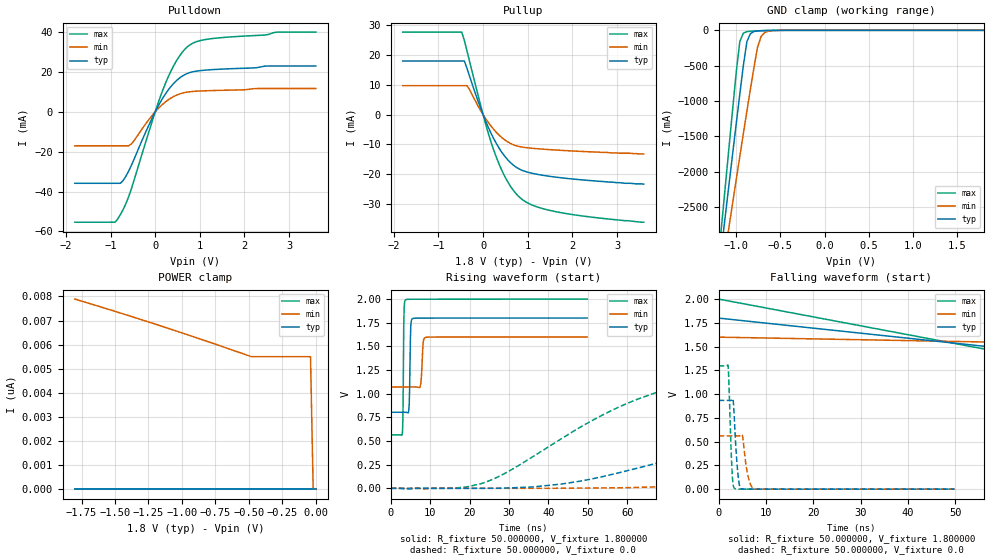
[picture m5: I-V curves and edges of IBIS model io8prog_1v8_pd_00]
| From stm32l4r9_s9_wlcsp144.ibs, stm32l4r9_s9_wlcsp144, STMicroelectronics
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|   Model io8prog_1v8_pd_00
[Model]  io8prog_1v8_pd_00
Model_type I/O
Polarity   Non-Inverting
Enable   Active-Low
Vinl =   0.540000V
Vinh =   1.260000V
Vmeas =  0.900000V
Cref =   100.000000nF
Rref =   1.000000k
Vref =   1.800000V
C_comp   2.197300pF   2.162700pF   2.264100pF
[Temperature Range]   25.000000   0.125000k   -40.000000
[Pullup Reference]   1.800000V   1.600000V   2.000000V
[Pulldown Reference]   0.0V   0.0V   0.0V
[POWER Clamp Reference]   1.800000V   1.600000V   2.000000V
[GND Clamp Reference]   0.0V   0.0V   0.0V
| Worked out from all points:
|   slope of the pulldown table from 0 to 0.27 V, typ, clamps not added: 26.2 ohm
|   slope of the pullup table from 0 to 0.27 V, typ, clamps not added: 30.1 ohm
|   GND clamp passes 1 mA (typ) near -0.58 V on its own axis
|   rising waveform, R_fixture 50.000000, V_fixture 1.800000: 20-80 % time 248ps typ, 382ps min, 184ps max; typ from 0.804 V to 1.8 V
|   rising waveform, R_fixture 50.000000, V_fixture 0.0: 20-80 % time 65.2ns typ, 116ns min, 36.2ns max; typ from 0 V to 0.933 V
|   falling waveform, R_fixture 50.000000, V_fixture 1.800000: 20-80 % time 115ns typ, 165ns min, 91.9ns max; typ from 1.8 V to 0.804 V
|   falling waveform, R_fixture 50.000000, V_fixture 0.0: 20-80 % time 709ps typ, 1.01ns min, 545ps max; typ from 0.933 V to 0 V
[Pulldown]
|Voltage   I(typ)   I(min)   I(max)
-1.8V     -35.82mA   -17.03mA   -55.34mA
-900mV    -35.82mA   -17.03mA   -55.34mA
-840mV    -35.82mA   -17.03mA   -53.76mA
-720mV    -34.49mA   -17.03mA   -49.08mA
-540mV    -27.18mA   -16.22mA   -39.07mA
-60mV     -2.756mA   -1.584mA   -4.226mA
240mV     9.353mA    5.172mA    14.85mA
480mV     15.75mA    8.427mA    25.77mA
720mV     19.29mA    9.947mA    32.62mA
960mV     20.57mA    10.43mA    35.5mA
1.32V     21.27mA    10.74mA    36.91mA
3.6V      23.03mA    11.73mA    40.05mA
[Pullup]
|Voltage   I(typ)   I(min)   I(max)
-1.8V     18.05mA    9.741mA    27.78mA
-480mV    18.05mA    9.741mA    27.78mA
-420mV    18.05mA    9.741mA    25.03mA
-360mV    15.57mA    9.741mA    21.38mA
60mV      -2.268mA   -1.401mA   -3.341mA
240mV     -8.143mA   -5.004mA   -12mA
360mV     -11.31mA   -6.914mA   -16.72mA
540mV     -15mA      -9.056mA   -22.31mA
840mV     -18.52mA   -10.83mA   -28.11mA
1.14V     -19.87mA   -11.38mA   -30.67mA
1.68V     -21.13mA   -11.96mA   -32.81mA
3.6V      -23.4mA    -13.2mA    -36.2mA
[GND_clamp]
|Voltage   I(typ)   I(min)   I(max)
-1.8V     -9.861A    -8.8A      -9.626A
-1.16V    -3.004A    -3.417A    -2.68A
-1.12V    -2.579A    -3.088A    -2.15A
-1.08V    -2.155A    -2.76A     -1.623A
-1V       -1.315A    -2.108A    -586.3mA
-960mV    -900.6mA   -1.784A    -158.3mA
-920mV    -496.8mA   -1.462A    -39.4mA
-880mV    -160.5mA   -1.144A    -17.83mA
-840mV    -45.94mA   -830.4mA   -12.53mA
-760mV    -8.275mA   -243mA     -7.558mA
-680mV    -3.402mA   -33.06mA   -3.844mA
1.8V      47.61uA    51.9uA     39.21uA
[POWER_clamp]
|Voltage   I(typ)   I(min)   I(max)
-1.8V     0A         7.891nA    0A
-1.14V    0A         6.744nA    0A
-480mV    0A         5.5nA      0A
-40mV     0A         5.5nA      0A
-20mV     0A         0A         0A
0V        0A         0A         0A
[Ramp]
| variable   typ   min   max
dV/dt_r  0.56009/65.12327n   0.33637/0.11606u   0.77826/36.16950n
dV/dt_f  0.59737/66.14891n   0.31692/0.11606u   0.86050/35.16380n
R_load = 50.000000
[Rising Waveform]
R_fixture= 50.000000
V_fixture= 1.800000
V_fixture_min= 1.600000
V_fixture_max= 2.000000
|time   V(typ)   V(min)   V(max)
0s        803.6mV    1.071V     565.2mV
2.903ns   803.6mV    1.071V     566.5mV
3.103ns   803.6mV    1.071V     740.3mV
3.403ns   803.6mV    1.071V     1.897V
3.804ns   803.4mV    1.071V     1.992V
4.605ns   827.4mV    1.071V     1.997V
5.105ns   1.718V     1.071V     1.997V
5.606ns   1.794V     1.071V     1.998V
8.809ns   1.798V     1.594V     1.998V
49.85ns   1.799V     1.599V     1.999V
[Rising Waveform]
R_fixture= 50.000000
V_fixture= 0.0
V_fixture_min= 0.0
V_fixture_max= 0.0
|time   V(typ)   V(min)   V(max)
0s        1.977nV    41.39nV    1.484nV
15.62ns   -76.86uV   -40.16uV   1.644mV
24.02ns   544.4uV    -30.84uV   64.54mV
43.24ns   44.68mV    938.1uV    522.3mV
55.26ns   138.3mV    4.907mV    806mV
73.27ns   327.9mV    21.32mV    1.086V
108.1ns   645.8mV    113.3mV    1.258V
157.4ns   852.3mV    285.6mV    1.292V
263.1ns   929mV      499.6mV    1.297V
598.2ns   933.5mV    560.6mV    1.297V
[Falling Waveform]
R_fixture= 50.000000
V_fixture= 1.800000
V_fixture_min= 1.600000
V_fixture_max= 2.000000
|time   V(typ)   V(min)   V(max)
0s        1.799V     1.599V     1.999V
150.2ns   1.006V     1.463V     593.7mV
300.3ns   816.7mV    1.135V     565.7mV
450.5ns   804.6mV    1.083V     565.3mV
750.8ns   803.6mV    1.071V     565.2mV
14.86us   803.6mV    1.071V     565.2mV
[Falling Waveform]
R_fixture= 50.000000
V_fixture= 0.0
V_fixture_min= 0.0
V_fixture_max= 0.0
|time   V(typ)   V(min)   V(max)
0s        933.5mV    560.6mV    1.297V
2.002ns   933.7mV    560.6mV    1.302V
2.803ns   937.5mV    560.7mV    226.5mV
3.103ns   927.7mV    560.8mV    37.93mV
3.403ns   666.3mV    560.9mV    6.923mV
4.204ns   103mV      560.5mV    481.7uV
4.805ns   4.882mV    573.6mV    137uV
6.306ns   123uV      118.5mV    54.06uV
7.508ns   1.644uV    2.567mV    38.57uV
49.85ns   1.977nV    41.39nV    1.484nV
